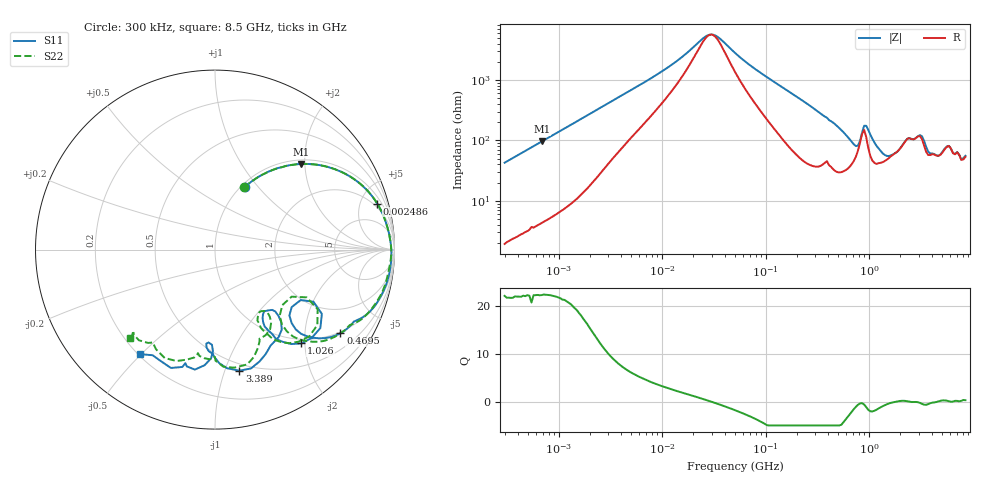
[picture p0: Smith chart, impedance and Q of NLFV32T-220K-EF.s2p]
! S-parameter Generated by TDK Corporation
! Copyright(C) 2015 TDK Corporation.
! All Rights Reserved.
! TDK P/N: NLFV32T-220K-EF (Inductors)
! Property: L=22uH at 2.52MHz
! Size(LxWxT): 3.2x2.5x2.2mm, 0.126x0.098x0.087inches
! Model Type: s2p (Touchstone File Format Version 1.0)
! Frequency: DC=Yes Start=0.3MHz Stop=8500MHz 225points Log-sweep
! Note:
! Model Generated on Jun. 23, 2015
! Hash(MD5):
! Port Assignments:
!  1 ---@@@--- 2
! Applicable Conditions:
!  Temperature = 25 degC
!  DC Bias Current = 0 A
!  Small Signal Operation
! Terms and conditions regarding TDK Simulation Models
! (1)This simulation model is being provided solely for informational purposes. Please refer to the specifications of the products in terms of detailed characteristics of such products.
! (2)In no event shall TDK Corporation of any of its subsidiaries be liable for any loss or damage arising, directly or indirectly,
!  From any information contained in this simulation model, including, but not limited to loss or damages arising from any inaccuracies, omissions or errors in connection with such information.
! (3)Any and all copyrights on this simulation model are owned by TDK Corporation.
!  Duplication or redistribution of this simulation model without prior written permission from TDK Corporation is prohibited.
! (4)This simulation model is subject to any modification or change without any prior notice.
! (5)Neither TDK Corporation nor any of its subsidiaries shall make any warranty, express or implied,
!  Including but not limited to the correctness, implied warranties of merchantability and fitness for a particular purpose with respect to this simulation models.
! (6)The use of this simulation model shall be deemed to have consented to the terms and conditions hereof.
# MHz S MA R 50
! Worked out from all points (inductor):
!   224 points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, 300 kHz to 8.5 GHz, reference 50 ohm
!   read as one part in series: L = 22.5 uH near 314.1 kHz
!   highest Q = 22.3 at 686.3 kHz (marker M1), where L = 22.2 uH
!   self-resonance near 29.53 MHz
!   S11 on the Smith chart (normalised r, x): 300 kHz: 1.04, +0.85; 2.486 MHz: 1.57, +6.83; 469.5 MHz: 0.95, -3.02; 1.026 GHz: 0.91, -1.93; 3.389 GHz: 0.44, -1.12; 8.5 GHz: 0.21, -0.49
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0.3  0.3853 64.7  0.9033 -22.7  0.9093 -22.9  0.3833 64.7
0.6862772  0.6765 44.8  0.7073 -42.6  0.7092 -42.9  0.6763 44.8
1.72111  0.9028 22.3  0.3817 -64.4  0.3829 -64.7  0.9036 22.3
2.486179  0.9394 15.8  0.2757 -69.5  0.2766 -69.9  0.9401 15.8
9.430415  0.9766 3.9  0.07464 -69.7  0.07472 -70.1  0.9765 3.8
28.42509  0.9828 -0.4  0.01759 -7.3  0.01761 -7.6  0.9819 -0.7
51.67171  0.9836 -2.8  0.03627 59.1  0.0363 58.8  0.9807 -3.2
283.1228  0.9395 -20.2  0.2629 63.0  0.2631 62.7  0.928 -21.7
469.456  0.84 -33.7  0.4297 45.8  0.43 45.4  0.825 -36.1
647.669  0.6717 -44.4  0.5642 25.5  0.5644 25.2  0.6492 -48.1
815.0429  0.5543 -30.5  0.4978 -1.7  0.4984 -1.9  0.5012 -31.5
893.5346  0.6948 -31.0  0.3606 5.4  0.3612 4.9  0.6615 -30.1
1025.67  0.7106 -47.3  0.4823 19.8  0.4814 19.4  0.6924 -47.8
1232.735  0.5695 -55.9  0.5934 6.3  0.594 5.8  0.5627 -57.9
1551.304  0.4493 -53.5  0.6078 -12.6  0.6082 -13.3  0.4451 -57.7
2044.041  0.482 -45.8  0.5207 -32.5  0.5211 -32.7  0.4558 -50.1
2346.313  0.5801 -50.1  0.431 -36.0  0.4311 -36.3  0.54 -55.4
3389.298  0.6881 -78.7  0.3935 -28.8  0.3929 -28.9  0.6664 -80.8
3890.506  0.5996 -90.3  0.4725 -39.3  0.4734 -39.9  0.5984 -90.0
4895.91  0.5188 -94.0  0.4622 -59.9  0.4635 -61.1  0.5845 -99.4
6161.135  0.6779 -99.5  0.3392 -68.5  0.3359 -68.7  0.6657 -114.9
8500  0.7175 -125.7  0.2791 -97.2  0.2789 -96.4  0.6838 -133.8
